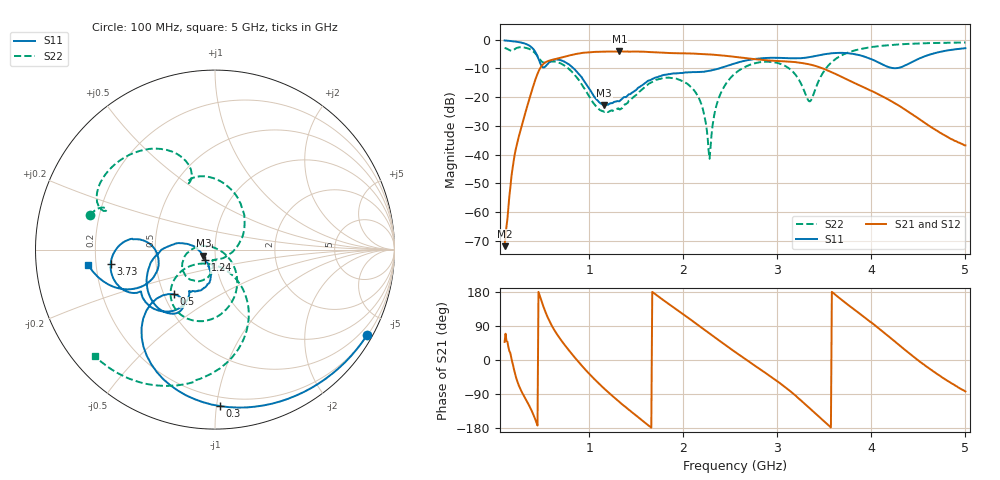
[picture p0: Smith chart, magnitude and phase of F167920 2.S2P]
!  2-Port S-parameters saved by WinCal
! VAR MeasName=S-Parameters (CALIBRATED_DATA) read from VNA (N5242A)
! VAR MeasDate=2016-11-22 9:53:30
! VAR NAME=F167920 2
! VAR FILENAME=F167920 2.S2P
! VAR DATE=2016-11-22 9:53:30
! VAR PHYS_PORTS=1,2
# Hz S DB R 50
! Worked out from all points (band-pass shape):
!   491 points, 100 MHz to 5 GHz, reference 50 ohm
!   highest |S21| = -4.06 dB at 1.32 GHz (marker M1); lowest = -71.8 dB at 100 MHz (marker M2)
!   |S21| within 3 dB of the highest: 598 MHz to 2.856 GHz (2.258 GHz wide, 131 % of centre)
!   lowest |S11| = -22.7 dB at 1.16 GHz (marker M3), VSWR 1.16, Z = 43.8 - j2.97 ohm
!   |S11| at or under -10 dB: 834.5 MHz to 2.378 GHz (1.543 GHz wide, 96.1 % of centre)
!   |S22| runs from -41.4 to -1.0 dB; largest |S21 - S12| = 0.0016
!   S11 on the Smith chart (normalised r, x): 100 MHz: 0.22, -3.82; 300 MHz: 0.14, -1.02; 500 MHz: 0.56, -0.32; 1.24 GHz: 0.89, -0.10; 3.73 GHz: 0.26, -0.06; 5 GHz: 0.17, -0.06
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1e8  -0.25 -29.3  -71.83 47.6  -70.36 77.4  -2.82 164.6
2e8  -0.58 -58.0  -41.41 -25.3  -41.33 -24.8  -3.45 160.6
3e8  -1.18 -88.1  -27.80 -92.2  -27.83 -92.2  -2.67 141.3
4.1e8  -3.45 -126.4  -15.57 -146.5  -15.56 -146.5  -4.19 115.9
5e8  -9.44 -132.4  -8.83 149.9  -8.83 150.0  -7.72 108.9
6.6e8  -6.87 -138.8  -6.57 66.9  -6.56 66.9  -7.79 95.6
9.2e8  -13.03 171.3  -4.60 -14.5  -4.59 -14.5  -15.57 24.4
1.16e9  -22.73 -152.5  -4.13 -75.7  -4.13 -75.7  -25.13 -77.5
1.24e9  -22.09 -133.7  -4.12 -93.3  -4.12 -93.3  -24.58 -97.3
1.32e9  -21.42 -119.2  -4.06 -110.2  -4.05 -110.2  -24.23 -104.0
1.74e9  -12.80 -107.2  -4.45 166.9  -4.44 166.9  -13.70 -122.7
2.12e9  -11.27 -122.0  -4.85 98.9  -4.84 98.9  -17.83 179.3
2.21e9  -11.18 -121.3  -5.01 82.7  -4.99 82.7  -24.37 159.7
2.28e9  -10.81 -119.9  -5.12 70.0  -5.11 70.0  -41.41 54.4
2.37e9  -10.08 -118.7  -5.33 53.6  -5.32 53.5  -21.01 -31.4
2.55e9  -8.21 -121.8  -5.95 21.3  -5.94 21.3  -11.75 -62.8
3.02e9  -6.30 -146.1  -7.44 -59.7  -7.42 -59.8  -8.26 -127.3
3.37e9  -5.89 -151.6  -8.79 -133.3  -8.76 -133.5  -20.29 -77.4
3.52e9  -4.95 -157.7  -10.46 -167.2  -10.44 -167.4  -9.86 -57.1
3.73e9  -4.63 -172.2  -13.64 149.7  -13.63 149.6  -4.73 -78.0
4.19e9  -9.59 -179.4  -20.98 61.1  -20.98 61.1  -1.87 -109.6
5e9  -2.95 -173.1  -36.75 -82.9  -36.83 -83.4  -0.97 -138.5
